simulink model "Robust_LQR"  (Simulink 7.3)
settings: Solver=ode45  StartTime=0.0  StopTime=80  RelTol=1e-3
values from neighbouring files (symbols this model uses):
  Cyb = -0.023    [init.m]    (also in init_lat.m; init_pitch.m)
  Cyda = 0.0011    [init.m]    (also in init_lat.m; init_pitch.m)
  Cydr = 0.0034    [init.m]    (also in init_lat.m; init_pitch.m)
  d2r = 1/r2d    (= 0.0174532925199)    [init.m]    (also in freq.m; frequ.m; init_lat.m; pl.m)
  Mv = 1219.1    [init.m]    (also in init_lat.m; init_pitch.m)
  Qbar = 1220.6    [init.m]    (also in init_lat.m; init_pitch.m)
  r2d = 180/pi    (= 57.2957795131)    [init.m]    (also in freq.m; frequ.m; init_lat.m; pl.m)
  Sref = 145.4    [init.m]    (also in init_lat.m; init_pitch.m)
undefined symbols (not defined in the file or in its folder): Avu, Bvu, Cvu, Dvu, Kpr

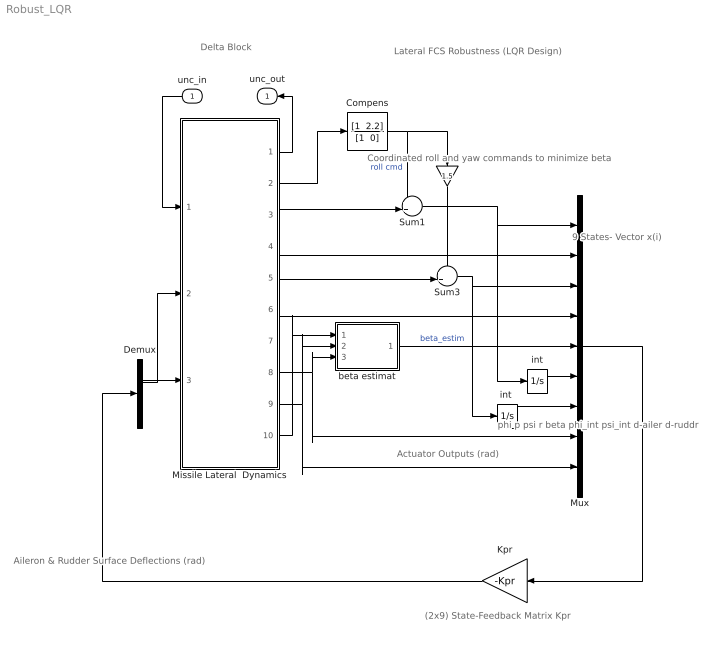
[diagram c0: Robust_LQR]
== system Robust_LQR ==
  note: phi p psi r beta phi_int psi_int d-ailer d-ruddr
  note: 9 States- Vector x(i)
  note: Aileron & Rudder Surface Deflections (rad)
  note: Actuator Outputs (rad)
  note: Coordinated roll and yaw commands to minimize beta
  note: (2x9) State-Feedback Matrix Kpr
  note: Lateral FCS Robustness (LQR Design)
  note: Delta Block
  unc_in : Inport  OutDataType=sfix(16)  OutScaling=2^0
  " " : Gain  Gain=1.5  ParameterDataType=fixdt(1, 16)  ParameterScaling=2^0  OutDataType=fixdt(1, 16)  OutScaling=2^0
  Compens : TransferFcn  Numerator="[1  2.2]"  Denominator="[1  0]"
  Demux : Demux  Outputs=2
  Kpr : Gain  Gain=-Kpr  Multiplication=Matrix(K*u)  ParameterDataType=fixdt(1, 16)  ParameterScaling=2^0  OutDataType=fixdt(1, 16)  OutScaling=2^0
  Missile Lateral  Dynamics : Subsystem
  Mux : Mux  Inputs=9
  Sum1 : Sum  Inputs=++|  OutDataType=fixdt(1, 16)  OutScaling=2^0
  Sum3 : Sum  Inputs=++|  OutDataType=fixdt(1, 16)  OutScaling=2^0
  beta estimat : Subsystem
  int : Integrator
  "int " : Integrator
  unc_out : Outport
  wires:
  Missile Lateral  Dynamics/8(dail) -> Mux/8, beta estimat/3(d-ail)
  Missile Lateral  Dynamics/9(drud) -> Mux/9, beta estimat/2(d-rud)
  Mux/1 -> Kpr/1
  Sum1/1 -> Mux/1, int/1
  int/1 -> Mux/6
  Compens/1 -> Sum1/1, " "/1  "roll cmd"
  Sum3/1 -> Mux/3, "int "/1
  "int "/1 -> Mux/7
  " "/1 -> Sum3/1
  Missile Lateral  Dynamics/2("Xi ") -> Compens/1
  Missile Lateral  Dynamics/3(phi) -> Sum1/2
  Missile Lateral  Dynamics/4(p) -> Mux/2
  Missile Lateral  Dynamics/5(psi) -> Sum3/2
  Missile Lateral  Dynamics/6(r) -> Mux/4
  Demux/1 -> Missile Lateral  Dynamics/2(ailer)
  Demux/2 -> Missile Lateral  Dynamics/3(rudd)
  Kpr/1 -> Demux/1
  beta estimat/1(beta) -> Mux/5  "beta_estim"
  Missile Lateral  Dynamics/10(Ny) -> beta estimat/1(Ny)
  Missile Lateral  Dynamics/1(unc_out) -> unc_out/1
  unc_in/1 -> Missile Lateral  Dynamics/1(unc_in)

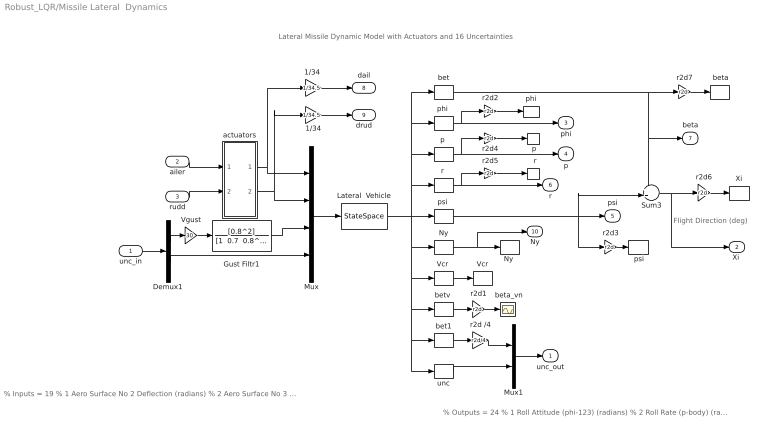
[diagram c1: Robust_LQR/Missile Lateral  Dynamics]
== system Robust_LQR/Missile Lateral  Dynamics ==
  note: Lateral Missile Dynamic Model with Actuators and 16 Uncertainties
  note: Flight Direction (deg)
  note: % Inputs = 19 % 1 Aero Surface No 2 Deflection (radians) % 2 Aero Surface No 3 Deflection (radians) % 3 Wind Gust Azim, Elev Angles=( 45.0 90.0) (deg) % 4 Cl_beta : -17.647 % Variation % 5 Cn_beta : 17.565 % Variation % 6 Cy_beta : -26.087 % Variation % 7 Cn_p : 36.023 % Variation % 8 Cn_r : -19.802 % Variation % 9 Cl_p : -20.576 % Variation % 10 Cl_r : 37.622 % Variation % 11 I_xx : 7.384 % Variation % 12 I_zz : 2.411 % Variation % 13 Xcg locat: 1.909 % Variation % 14 Cy_surf 2: 45.455 % Variation % 15 Cl_surf 2: -15.289 % Variation % 16 Cn_surf 2: -28.571 % Variation % 17 Cy_surf 3: 29.412 % Variation % 18 Cl_surf 3: 16.819 % Variation % 19 Cn_surf 3: -28.571 % Variation
  note: % Outputs = 24 % 1 Roll Attitude (phi-123) (radians) % 2 Roll Rate (p-body) (rad/sec) % 3 Yaw Attitude (psi-123) (radians) % 4 Yaw Rate (r-body) (rad/sec) % 5 Angle of sideslip, beta, (radian) % 6 Cross Range Velocity (Vcr) (ft/sec) % 7 Accelerom # 1, (along Y), (ft/sec^2) % 8 Beta Sensed at Vane # 1 (radian) % 9 Cl_beta : -17.647 % Variation % 10 Cn_beta : 17.565 % Variation % 11 Cy_beta : -26.087 % Variation % 12 Cn_p : 36.023 % Variation % 13 Cn_r : -19.802 % Variation % 14 Cl_p : -20.576 % Variation % 15 Cl_r : 37.622 % Variation % 16 I_xx : 7.384 % Variation % 17 I_zz : 2.411 % Variation % 18 Xcg locat: 1.909 % Variation % 19 Cy_surf 2: 45.455 % Variation % 20 Cl_surf 2: -15.289 % Variation % 21 Cn_surf 2: -28.571 % Variation % 22 Cy_surf 3: 29.412 % Variation % 23 Cl_surf 3: 16.819 % Variation % 24 Cn_surf 3: -28.571 % Variation
  unc_in : Inport  OutDataType=sfix(16)  OutScaling=2^0
  ailer : Inport  Port=2  OutDataType=sfix(16)  OutScaling=2^0
  rudd : Inport  Port=3  OutDataType=sfix(16)  OutScaling=2^0
  "  r" : ToWorkspace  VariableName=r  SampleTime=-1  SaveFormat=Array
  " Ny " : Selector  InputPortWidth=24  IndexOptions=Index vector (dialog)  Indices=[7]  OutputSizes=1
  " Xi " : ToWorkspace  VariableName=Xi  SampleTime=-1  SaveFormat=Array
  " beta" : ToWorkspace  VariableName=beta  SampleTime=-1  SaveFormat=Array
  " beta_vn" : Scope
  " p" : ToWorkspace  VariableName=p  SampleTime=-1  SaveFormat=Array
  " phi " : ToWorkspace  VariableName=phi  SampleTime=-1  SaveFormat=Array
  " psi" : ToWorkspace  VariableName=psi  SampleTime=-1  SaveFormat=Array
  1/34 : Gain  Gain=1/34.5  ParameterDataType=fixdt(1, 16)  ParameterScaling=2^0  OutDataType=fixdt(1, 16)  OutScaling=2^0
  "1/34 " : Gain  Gain=1/34.5  ParameterDataType=fixdt(1, 16)  ParameterScaling=2^0  OutDataType=fixdt(1, 16)  OutScaling=2^0
  Demux1 : Demux  Outputs=[1, 16]
  Gust Filtr1 : TransferFcn  Numerator=[0.8^2]  Denominator="[1  0.7  0.8^2]"
  Lateral  Vehicle : StateSpace  A=Avu  B=Bvu  C=Cvu  D=Dvu
  Mux : Mux  Inputs=[1, 1, 1, 16]
  Mux1 : Mux  Inputs="[1,  16]"
  "Ny " : ToWorkspace  VariableName=Ny  SampleTime=-1  SaveFormat=Array
  Sum3 : Sum  Inputs=++|  OutDataType=fixdt(1, 16)  OutScaling=2^0
  Vcr : ToWorkspace  VariableName=Vcr  SampleTime=-1  SaveFormat=Array
  "Vcr " : Selector  InputPortWidth=24  IndexOptions=Index vector (dialog)  Indices=[6]  OutputSizes=1
  Vgust : Gain  Gain=30  ParameterDataType=fixdt(1, 16)  ParameterScaling=2^0  OutDataType=fixdt(1, 16)  OutScaling=2^0
  actuators : Subsystem
  bet : Selector  InputPortWidth=24  IndexOptions=Index vector (dialog)  Indices=[5]  OutputSizes=1
  bet1 : Selector  InputPortWidth=24  IndexOptions=Index vector (dialog)  Indices=[5]  OutputSizes=1
  "betv " : Selector  InputPortWidth=24  IndexOptions=Index vector (dialog)  Indices=[8]  OutputSizes=1
  "p " : Selector  InputPortWidth=24  IndexOptions=Index vector (dialog)  Indices=[2]  OutputSizes=1
  "phi " : Selector  InputPortWidth=24  IndexOptions=Index vector (dialog)  Indices=[1]  OutputSizes=1
  "psi " : Selector  InputPortWidth=24  IndexOptions=Index vector (dialog)  Indices=[3]  OutputSizes=1
  "r " : Selector  InputPortWidth=24  IndexOptions=Index vector (dialog)  Indices=[4]  OutputSizes=1
  r2d /4 : Gain  Gain=r2d/4  ParameterDataType=fixdt(1, 16)  ParameterScaling=2^0  OutDataType=fixdt(1, 16)  OutScaling=2^0
  r2d{1..7} (7 alike) : Gain  Gain=r2d  ParameterDataType=fixdt(1, 16)  ParameterScaling=2^0  OutDataType=fixdt(1, 16)  OutScaling=2^0
  unc : Selector  InputPortWidth=24  IndexOptions=Index vector (dialog)  Indices=[9:24]  OutputSizes=1
  unc_out : Outport
  "Xi " : Outport  Port=2
  phi : Outport  Port=3
  p : Outport  Port=4
  psi : Outport  Port=5
  r : Outport  Port=6
  beta : Outport  Port=7
  dail : Outport  Port=8  OutDataType=sfix(16)  OutScaling=2^0
  drud : Outport  Port=9  OutDataType=sfix(16)  OutScaling=2^0
  Ny : Outport  Port=10
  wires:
  Mux/1 -> Lateral  Vehicle/1
  ailer/1 -> actuators/1(da)
  rudd/1 -> actuators/2(dr)
  Lateral  Vehicle/1 -> bet/1, "phi "/1, "p "/1, "r "/1, "betv "/1, unc/1, bet1/1, "Vcr "/1, " Ny "/1, "psi "/1
  actuators/1("da ") -> Mux/1, "1/34 "/1
  actuators/2("dr ") -> Mux/2, 1/34/1
  1/34/1 -> drud/1
  "1/34 "/1 -> dail/1
  Sum3/1 -> "Xi "/1, r2d6/1
  r2d1/1 -> " beta_vn"/1
  r2d6/1 -> " Xi "/1
  r2d3/1 -> " psi"/1
  r2d2/1 -> " phi "/1
  r2d4/1 -> " p"/1
  r2d5/1 -> "  r"/1
  r2d7/1 -> " beta"/1
  bet/1 -> Sum3/1, beta/1, r2d7/1
  "phi "/1 -> phi/1, r2d2/1
  "p "/1 -> r2d4/1, p/1
  "r "/1 -> r/1, r2d5/1
  "psi "/1 -> Sum3/2, psi/1, r2d3/1
  " Ny "/1 -> "Ny "/1, Ny/1
  "Vcr "/1 -> Vcr/1
  "betv "/1 -> r2d1/1
  bet1/1 -> r2d /4/1
  unc/1 -> Mux1/2
  Mux1/1 -> unc_out/1
  Demux1/1 -> Vgust/1
  Demux1/2 -> Mux/4
  Vgust/1 -> Gust Filtr1/1
  Gust Filtr1/1 -> Mux/3
  unc_in/1 -> Demux1/1
  r2d /4/1 -> Mux1/1

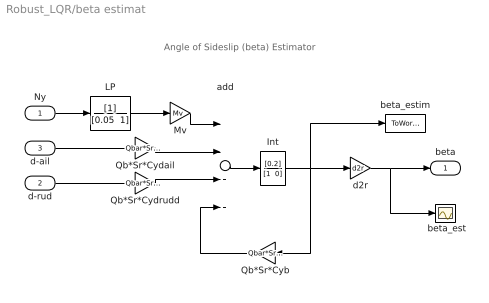
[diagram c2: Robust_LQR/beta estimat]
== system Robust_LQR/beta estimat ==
  note: Angle of Sideslip (beta) Estimator
  Ny : Inport
  d-rud : Inport  Port=2
  d-ail : Inport  Port=3
  " beta_est" : Scope
  Int : TransferFcn  Numerator=[0.2]  Denominator="[1  0]"
  LP : TransferFcn  Denominator="[0.05  1]"
  Mv : Gain  Gain=Mv  ParameterDataType=fixdt(1, 16)  ParameterScaling=2^0  OutDataType=fixdt(1, 16)  OutScaling=2^0
  Qb*Sr*Cyb : Gain  Gain=Qbar*Sref*Cyb*1.2  ParameterDataType=fixdt(1, 16)  ParameterScaling=2^0  OutDataType=fixdt(1, 16)  OutScaling=2^0
  Qb*Sr*Cydail : Gain  Gain=Qbar*Sref*Cyda*34  ParameterDataType=fixdt(1, 16)  ParameterScaling=2^0  OutDataType=fixdt(1, 16)  OutScaling=2^0
  Qb*Sr*Cydrudd : Gain  Gain=Qbar*Sref*Cydr*34  ParameterDataType=fixdt(1, 16)  ParameterScaling=2^0  OutDataType=fixdt(1, 16)  OutScaling=2^0
  add : Sum  Inputs=-+++  OutDataType=fixdt(1, 16)  OutScaling=2^-10
  beta_estim : ToWorkspace  VariableName=beta_vn  SampleTime=-1  SaveFormat=Array
  d2r : Gain  Gain=d2r  ParameterDataType=fixdt(1, 16)  ParameterScaling=2^0  OutDataType=fixdt(1, 16)  OutScaling=2^0
  beta : Outport
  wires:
  add/1 -> Int/1
  Mv/1 -> add/1
  d2r/1 -> " beta_est"/1, beta/1
  Int/1 -> Qb*Sr*Cyb/1, d2r/1, beta_estim/1
  d-ail/1 -> Qb*Sr*Cydail/1
  Ny/1 -> LP/1
  d-rud/1 -> Qb*Sr*Cydrudd/1
  Qb*Sr*Cyb/1 -> add/4
  Qb*Sr*Cydrudd/1 -> add/3
  Qb*Sr*Cydail/1 -> add/2
  LP/1 -> Mv/1

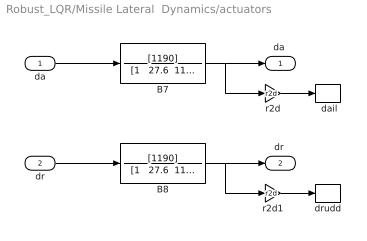
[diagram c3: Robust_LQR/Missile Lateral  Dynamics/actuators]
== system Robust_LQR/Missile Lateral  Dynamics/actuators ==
  da : Inport
  dr : Inport  Port=2
  " dail" : ToWorkspace  VariableName=dail  SampleTime=-1  SaveFormat=Array
  " drudd " : ToWorkspace  VariableName=drud  SampleTime=-1  SaveFormat=Array
  B7 : TransferFcn  Numerator=[1190]  Denominator="[1   27.6  1190]"
  B8 : TransferFcn  Numerator=[1190]  Denominator="[1   27.6  1190]"
  r2d : Gain  Gain=r2d  ParameterDataType=fixdt(1, 16)  ParameterScaling=2^0  OutDataType=fixdt(1, 16)  OutScaling=2^0
  r2d1 : Gain  Gain=r2d  ParameterDataType=fixdt(1, 16)  ParameterScaling=2^0  OutDataType=fixdt(1, 16)  OutScaling=2^0
  "da " : Outport
  "dr " : Outport  Port=2
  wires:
  B8/1 -> "dr "/1, r2d1/1
  dr/1 -> B8/1
  B7/1 -> "da "/1, r2d/1
  da/1 -> B7/1
  r2d1/1 -> " drudd "/1
  r2d/1 -> " dail"/1
